PROGRAM MAIN
VAR
	fDutyCycle			:	REAL := 50.0	;		(*占空比 ：0%到100%*)
	fFrequency			:	REAL := 1000.0	;		(*时钟频率 ：15.26Hz 到 100kHz*)
	nOutput		AT %Q*	:	UINT 			;
	nPeriod		AT %Q*	:	UINT			;
	
END_VAR

nOutput := REAL_TO_UINT (fDutyCycle/100*65535);
nPeriod := REAL_TO_UINT (1/fFrequency*1000000);

END_PROGRAM
